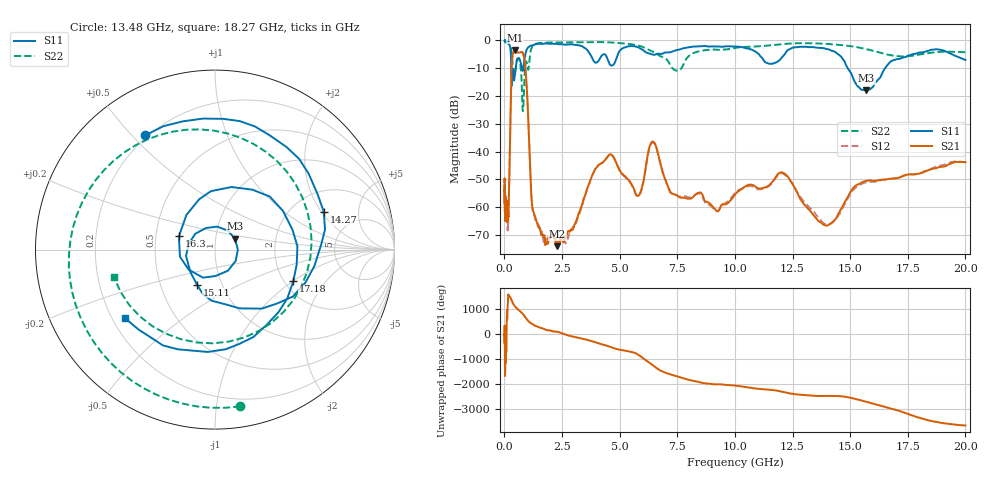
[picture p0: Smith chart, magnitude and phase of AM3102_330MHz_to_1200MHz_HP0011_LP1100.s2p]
! Date/Time: Tue, Sep 11, 2018 5:12 PM
! Network Analyzer: Agilent Technologies E8362B Rev: A.07.50.63
! Sweep from 0.010 to 20.000 GHz, 1601 Points, Sweep Type: LOG
! Power Supply: 4.949 V, 0.001 A
# Hz S DB R 50
!freq MagS11 AngS11 MagS21 AngS21 MagS12 AngS12 MagS22 AngS22
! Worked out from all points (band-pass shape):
!   1601 points, 10 MHz to 20 GHz, reference 50 ohm
!   highest |S21| = -3.40 dB at 458 MHz (marker M1); lowest = -74.1 dB at 2.303 GHz (marker M2)
!   |S21| within 3 dB of the highest: 340.8 MHz to 858.7 MHz (517.9 MHz wide, 86.4 % of centre)
!   lowest |S11| = -18.0 dB at 15.7 GHz (marker M3), VSWR 1.29, Z = 62 + j7.63 ohm
!   |S11| at or under -10 dB: 298.9 MHz to 496.1 MHz (197.2 MHz wide, 49.6 % of centre); 756.7 MHz to 823 MHz (66.33 MHz wide, 8.4 % of centre); 14.89 GHz to 16.52 GHz (1.621 GHz wide, 10.3 % of centre)
!   |S22| runs from -25.4 to -0.3 dB; largest |S21 - S12| = 0.012
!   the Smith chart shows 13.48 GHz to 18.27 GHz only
!   S11 on the Smith chart (normalised r, x): 13.48 GHz: 0.19, +0.54; 14.27 GHz: 2.96, +2.11; 15.11 GHz: 0.76, -0.31; 16.3 GHz: 0.66, +0.10; 17.18 GHz: 2.23, -1.01; 18.27 GHz: 0.25, -0.32
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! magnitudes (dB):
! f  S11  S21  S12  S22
! 10 MHz  0.0  -50.2  -49.9  -0.3
! 35.55 MHz  0.0  -59.7  -60.9  -0.5
! 126.4 MHz  -0.4  -65.5  -61.8  -1.0
! 177.9 MHz  -0.9  -61.0  -62.5  -1.2
! 313.2 MHz  -15.5  -9.9  -9.9  -5.1
! 447.2 MHz  -13.1  -3.4  -3.5  -11.7
! 458 MHz  -12.5  -3.4  -3.4  -11.3
! 873.8 MHz  -6.7  -7.2  -7.3  -12.8
! 1.207 GHz  -1.8  -59.7  -60.2  -2.2
! 1.59 GHz  -1.3  -69.6  -68.6  -0.9
! 2.303 GHz  -1.3  -74.1  -73.4  -0.7
! 4.521 GHz  -7.7  -41.4  -41.3  -0.7
! 5.652 GHz  -2.1  -54.2  -54.6  -1.6
! 6.457 GHz  -5.2  -36.5  -36.8  -4.1
! 13.48 GHz  -2.5  -63.6  -62.3  -1.1
! 14.27 GHz  -3.9  -65.1  -65.3  -1.4
! 15.11 GHz  -13.2  -53.3  -54.0  -2.2
! 15.7 GHz  -18.0  -50.6  -51.1  -3.1
! 16.3 GHz  -13.4  -50.2  -50.4  -4.4
! 17.18 GHz  -6.5  -49.2  -49.1  -5.7
! 18.27 GHz  -4.0  -47.1  -47.0  -4.7
! 20 GHz  -7.1  -43.8  -43.9  -4.2
